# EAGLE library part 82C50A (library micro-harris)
MICROCONTROLLER/MEMORY DEVICE
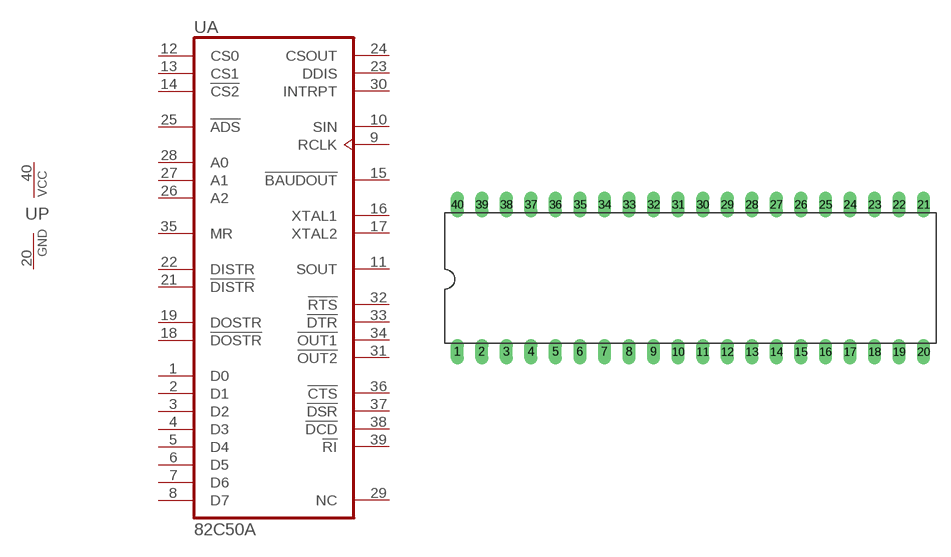
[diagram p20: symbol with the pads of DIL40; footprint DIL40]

Designator prefix U; gates A=82C50A P=PWRN

## 82C50A (MPN: CP82C50A-5; OC_FARNELL: 527750; OC_NEWARK: 06F3286)  [DIL40]
1  A:D0
2  A:D1
3  A:D2
4  A:D3
5  A:D4
6  A:D5
7  A:D6
8  A:D7
9  A:RCLK  in
10  A:SIN  in
11  A:SOUT  out
12  A:CS0  in
13  A:CS1  in
14  A:!CS2  in
15  A:!BAUDOUT  out
16  A:XTAL1  in
17  A:XTAL2  out
18  A:!DOSTR  in
19  A:DOSTR  in
20  P:GND  pwr
21  A:!DISTR  in
22  A:DISTR  in
23  A:DDIS  out
24  A:CSOUT  out
25  A:!ADS  in
26  A:A2  in
27  A:A1  in
28  A:A0  in
29  A:NC  nc
30  A:INTRPT  out
31  A:!OUT2  out
32  A:!RTS  out
33  A:!DTR  out
34  A:!OUT1  out
35  A:MR  in
36  A:!CTS  in
37  A:!DSR  in
38  A:!DCD  in
39  A:!RI  in
40  P:VCC  pwr

## Footprint DIL40 (pad centres in mm)
Dual In Line Package
drill 0.813 long: 1 -24.13,-7.62; 2 -21.59,-7.62; 3 -19.05,-7.62; 4 -16.51,-7.62; 5 -13.97,-7.62; 6 -11.43,-7.62; 7 -8.89,-7.62; 8 -6.35,-7.62; 9 -3.81,-7.62; 10 -1.27,-7.62; 11 1.27,-7.62; 12 3.81,-7.62; 13 6.35,-7.62; 14 8.89,-7.62; 15 11.43,-7.62; 16 13.97,-7.62; 17 16.51,-7.62; 18 19.05,-7.62; 19 21.59,-7.62; 20 24.13,-7.62; 21 24.13,7.62; 22 21.59,7.62; 23 19.05,7.62; 24 16.51,7.62; 25 13.97,7.62; 26 11.43,7.62; 27 8.89,7.62; 28 6.35,7.62; 29 3.81,7.62; 30 1.27,7.62; 31 -1.27,7.62; 32 -3.81,7.62; 33 -6.35,7.62; 34 -8.89,7.62; 35 -11.43,7.62; 36 -13.97,7.62; 37 -16.51,7.62; 38 -19.05,7.62; 39 -21.59,7.62; 40 -24.13,7.62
